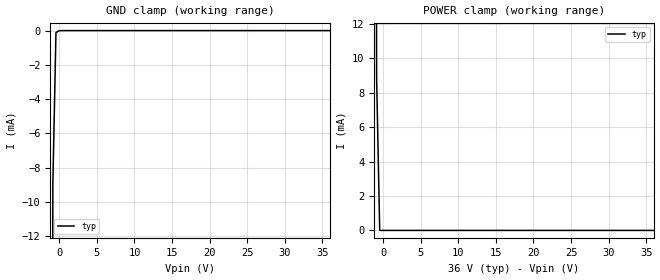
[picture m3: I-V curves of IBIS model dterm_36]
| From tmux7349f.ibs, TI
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| dterm_36
[Model]   dterm_36
Model_type   Terminator
|   typ   min   max
C_comp   1.008417e-11   NA   NA
[Voltage Range]   36   NA   NA
[Temperature Range]   27   NA   NA
[Power Clamp Reference]   36   NA   NA
[GND Clamp Reference]   0   NA   NA
[GND Clamp]
|   Voltage   I(typ)   I(min)   I(max)
-5V       -1.414A    NA         NA
-1.273V   -125.7mA   NA         NA
-858.6mV  -8.97mA    NA         NA
-444.4mV  -116uA     NA         NA
-30.3mV   -7.891uA   NA         NA
383.8mV   -5.778nA   NA         NA
36V       7.24nA     NA         NA
[POWER Clamp]
|   Voltage   I(typ)   I(min)   I(max)
-5V       1.414A     NA         NA
-1.273V   125.5mA    NA         NA
-858.6mV  8.924mA    NA         NA
-444.4mV  50.58nA    NA         NA
36V       -4.424uA   NA         NA
